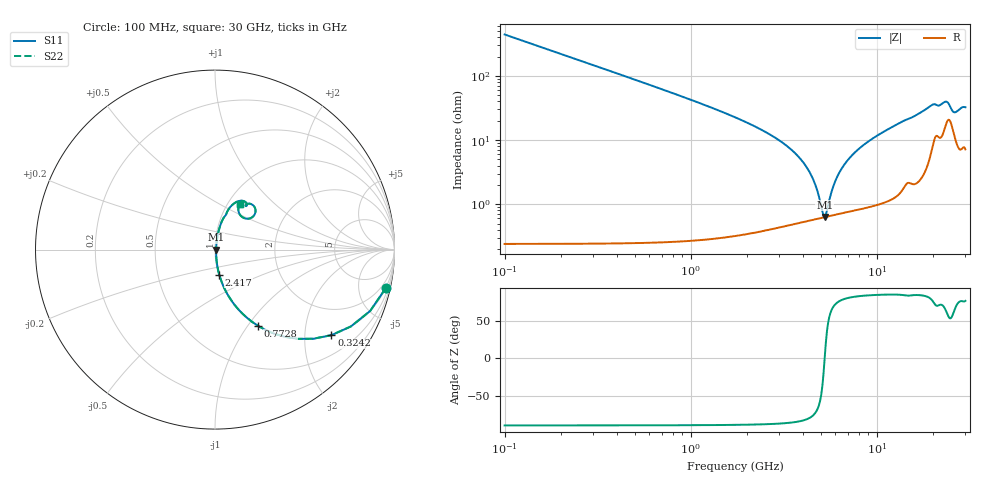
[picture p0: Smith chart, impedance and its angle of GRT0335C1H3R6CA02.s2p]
!Murata Part Number: GRT0335C1H3R6CA02
!These Parameters are Measured in Series Mode Connection
!Data Generated on Jun 19, 2026
!  o--ll--o
!Port1  Port2
!  o------o
!Operation Temp=25[degC], DC Bias Voltage=0[V]
!Freq. Start=100[MHz] Stop=30[GHz] 401[Steps]
# Hz S RI R 50
!Freq.(Hz) S11(Real) S11(Imag) S21(Real) S21(Imag) S12(Real) S12(Imag) S22(Real) S22(Imag)
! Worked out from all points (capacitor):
!   401 points, 100 MHz to 30 GHz, reference 50 ohm
!   read as one part in series: C = 3.6 pF near 249.5 MHz
!   lowest |Z| = 631 mohm at 5.258 GHz (marker M1)
!   series resonance near 5.254 GHz, so ESL is about 250 pH
!   S11 on the Smith chart (normalised r, x): 100 MHz: 1.00, -8.84; 324.2 MHz: 1.00, -2.72; 772.8 MHz: 1.01, -1.12; 2.417 GHz: 1.01, -0.29; 30 GHz: 1.14, +0.63
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1e8  0.9512 -0.2152  0.0488 0.2152  0.0488 0.2152  0.9512 -0.2152
3.2425e8  0.6482 -0.4766  0.3518 0.4766  0.3518 0.4766  0.6482 -0.4766
5.485e8  0.3887 -0.4859  0.6113 0.4859  0.6113 0.4859  0.3887 -0.4859
7.7275e8  0.2393 -0.4243  0.7607 0.4243  0.7607 0.4243  0.2393 -0.4243
1.37075e9  0.0847 -0.2736  0.9153 0.2736  0.9153 0.2736  0.0847 -0.2736
2.41725e9  0.0237 -0.1393  0.9763 0.1393  0.9763 0.1393  0.0237 -0.1393
3.5385e9  0.0093 -0.0666  0.9907 0.0666  0.9907 0.0666  0.0093 -0.0666
4.21125e9  0.00677 -0.0366  0.9932 0.0366  0.9932 0.0366  0.00677 -0.0366
4.65975e9  0.00619 -0.0197  0.9938 0.0197  0.9938 0.0197  0.00619 -0.0197
5.10825e9  0.00618 -0.00461  0.9938 0.00461  0.9938 0.00461  0.00618 -0.00461
5.25775e9  0.00627 0.000121  0.9937 -0.000121  0.9937 -0.000121  0.00627 0.000121
5.40725e9  0.00641 0.00471  0.9936 -0.00471  0.9936 -0.00471  0.00641 0.00471
6.00525e9  0.0073 0.0219  0.9927 -0.0219  0.9927 -0.0219  0.0073 0.0219
6.75275e9  0.00907 0.0414  0.9909 -0.0414  0.9909 -0.0414  0.00907 0.0414
8.09825e9  0.0136 0.0726  0.9864 -0.0726  0.9864 -0.0726  0.0136 0.0726
1.01165e10  0.023 0.1141  0.977 -0.1141  0.977 -0.1141  0.023 0.1141
1.505e10  0.0628 0.1982  0.9372 -0.1982  0.9372 -0.1982  0.0628 0.1982
2.005825e10  0.1629 0.2692  0.8371 -0.2692  0.8371 -0.2692  0.1629 0.2692
2.35715e10  0.22 0.2375  0.78 -0.2375  0.78 -0.2375  0.22 0.2375
2.50665e10  0.193 0.1736  0.807 -0.1736  0.807 -0.1736  0.193 0.1736
2.618775e10  0.1447 0.1873  0.8553 -0.1873  0.8553 -0.1873  0.1447 0.1873
3e10  0.1417 0.2534  0.8583 -0.2534  0.8583 -0.2534  0.1417 0.2534
